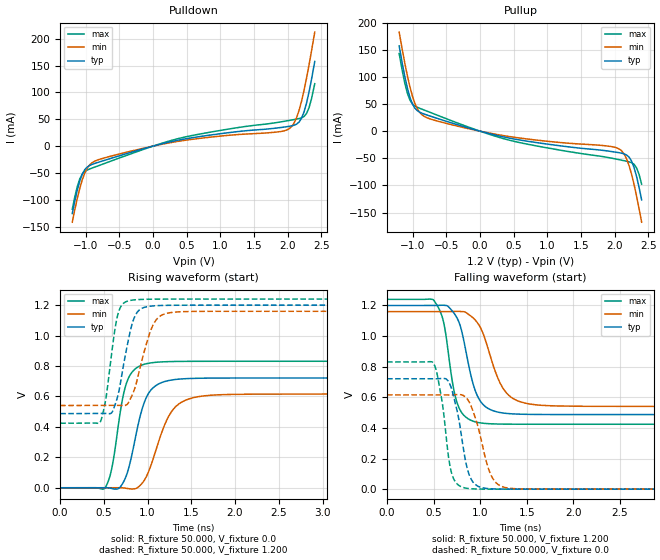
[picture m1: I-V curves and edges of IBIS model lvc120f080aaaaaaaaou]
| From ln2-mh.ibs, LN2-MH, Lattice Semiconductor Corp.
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|   Model lvc120f080aaaaaaaaou
[Model] lvc120f080aaaaaaaaou
Model_type Output
Polarity   Non-Inverting
Enable   Active-High
Vmeas =  0.600V
Cref =  0.0F
Rref =  1.000M
Vref =  0.0V
C_comp   5.000pF   4.000pF   5.500pF
[Temperature Range]   25.000   0.125k   -40.000
[Voltage Range]   1.200V   1.160V   1.240V
[C Comp Corner]
C_comp   5.000pF   4.000pF   5.500pF
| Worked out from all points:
|   slope of the pulldown table from 0 to 0.18 V, typ, clamps not added: 31.3 ohm
|   slope of the pullup table from 0 to 0.18 V, typ, clamps not added: 31.2 ohm
|   rising waveform, R_fixture 50.000, V_fixture 0.0: 20-80 % time 183ps typ, 243ps min, 143ps max; typ from 0 V to 0.721 V
|   rising waveform, R_fixture 50.000, V_fixture 1.200: 20-80 % time 144ps typ, 178ps min, 114ps max; typ from 0.487 V to 1.2 V
|   falling waveform, R_fixture 50.000, V_fixture 1.200: 20-80 % time 165ps typ, 222ps min, 128ps max; typ from 1.2 V to 0.487 V
|   falling waveform, R_fixture 50.000, V_fixture 0.0: 20-80 % time 131ps typ, 163ps min, 107ps max; typ from 0.721 V to 0 V
[Pulldown]
|Voltage   I(typ)   I(min)   I(max)
-1.2V     -125.5mA   -141.7mA   -117.5mA
-1.126V   -82.18mA   -97.71mA   -75.64mA
-1.052V   -52.35mA   -62.95mA   -52.09mA
-978mV    -38.99mA   -41.1mA    -44.58mA
-867mV    -32.34mA   -28.12mA   -39.09mA
391mV     11.49mA    9.231mA    14.53mA
2.019V    36.8mA     32.22mA    47.75mA
2.13V     40.84mA    52.82mA    50.28mA
2.204V    51.83mA    83.7mA     52.6mA
2.278V    80.16mA    126.5mA    60.63mA
2.315V    100.7mA    151.1mA    71.46mA
2.4V      157.6mA    212.3mA    116.2mA
[Pullup]
|Voltage   I(typ)   I(min)   I(max)
-1.2V     157.2mA    182.6mA    143.1mA
-1.115V   100.2mA    124.6mA    87.96mA
-1.041V   62.63mA    82.08mA    57.47mA
-967mV    42.4mA     51.3mA     46.5mA
-856mV    32.8mA     29.67mA    40.24mA
-412mV    14.79mA    11.57mA    18.71mA
439mV     -12.88mA   -9.955mA   -16.74mA
2.067V    -39.79mA   -32.82mA   -52.62mA
2.178V    -44.03mA   -51.4mA    -55.48mA
2.252V    -55.53mA   -80.14mA   -58.17mA
2.326V    -84.03mA   -120.3mA   -67.92mA
2.4V      -126.7mA   -167.8mA   -97.74mA
[Ramp]
| variable   typ   min   max
dV/dt_r   0.433/0.183n   0.370/0.243n   0.499/0.143n
dV/dt_f   0.428/0.165n   0.372/0.222n   0.490/0.129n
R_load = 50.000
[Rising Waveform]
R_fixture= 50.000
V_fixture= 0.0
V_fixture_min= 0.0
V_fixture_max= 0.0
|time   V(typ)   V(min)   V(max)
0s        20.81nV    937.6nV    2.143nV
513ps     229.8uV    -23.32uV   -1.57mV
589ps     -4.804mV   42.42uV    123.7mV
679ps     -344.7uV   249.6uV    465.2mV
797ps     158.5mV    -7.184mV   738.4mV
929ps     500.9mV    23.81mV    805mV
1.043ns   645.5mV    155mV      821mV
1.296ns   709.9mV    517.2mV    829.6mV
1.716ns   720.5mV    607.6mV    831.1mV
10ns      721.4mV    615.9mV    831.2mV
[Rising Waveform]
R_fixture= 50.000
V_fixture= 1.200
V_fixture_min= 1.160
V_fixture_max= 1.240
|time   V(typ)   V(min)   V(max)
0s        487.4mV    540.6mV    424.1mV
456ps     488.5mV    541.2mV    429.4mV
521ps     488.3mV    541.4mV    578.8mV
594ps     496.6mV    541.6mV    906.1mV
658ps     600.7mV    541.5mV    1.135V
826ps     1.082V     612.4mV    1.233V
906ps     1.168V     769.9mV    1.237V
1.065ns   1.195V     1.072V     1.239V
1.305ns   1.199V     1.154V     1.24V
10ns      1.2V       1.16V      1.24V
[Falling Waveform]
R_fixture= 50.000
V_fixture= 1.200
V_fixture_min= 1.160
V_fixture_max= 1.240
|time   V(typ)   V(min)   V(max)
0s        1.2V       1.16V      1.24V
497ps     1.2V       1.16V      1.237V
601ps     1.202V     1.16V      1.106V
666ps     1.188V     1.16V      851.7mV
783ps     1.072V     1.161V     518.6mV
922ps     691.2mV    1.12V      444.6mV
1.01ns    568mV      1.046V     432.3mV
1.262ns   496.3mV    643.6mV    424.9mV
1.589ns   488.2mV    551.5mV    424.2mV
10ns      487.3mV    540.6mV    424.1mV
[Falling Waveform]
R_fixture= 50.000
V_fixture= 0.0
V_fixture_min= 0.0
V_fixture_max= 0.0
|time   V(typ)   V(min)   V(max)
0s        721.4mV    615.9mV    831.2mV
495ps     721.1mV    615.9mV    825.5mV
585ps     723mV      615.8mV    593.7mV
691ps     658.4mV    615.7mV    109mV
763ps     480.2mV    618mV      28.2mV
866ps     123.7mV    584.7mV    4.981mV
955ps     27.02mV    451.1mV    1.298mV
1.119ns   2.511mV    87.55mV    188.6uV
1.328ns   282.1uV    5.168mV    41.66uV
10ns      4.084uV    8.864uV    1.884uV
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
